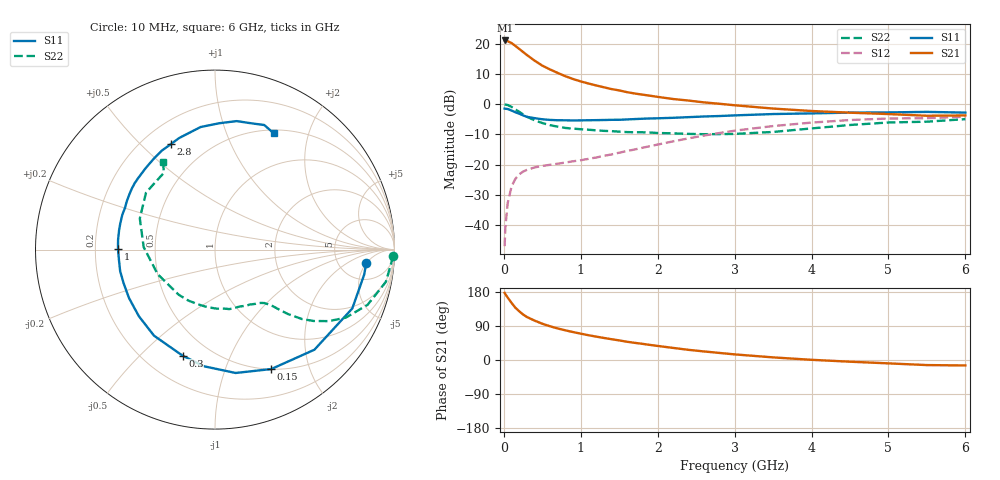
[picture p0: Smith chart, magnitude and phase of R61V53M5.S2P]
! SIEMENS Small Signal Semiconductors
! BFR193
! Si NPN RF Bipolar Junction Transistor in SOT23
! VCE = 1.5 V  IC = 3.5 mA
! Common Emitter S-Parameters:  May  1996
# GHz  S  MA  R  50
!  f  S11  S21  S12  S22
! GHz  MAG  ANG  MAG  ANG  MAG  ANG  MAG  ANG
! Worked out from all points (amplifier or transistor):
!   36 points, 10 MHz to 6 GHz, reference 50 ohm
!   highest |S21| = 21.1 dB at 20 MHz (marker M1)
!   |S21| within 3 dB of that: start of sweep to 209.9 MHz
!   unconditionally stable (mu >= 1): 985.2 MHz to 2.083 GHz
!   at 250 MHz: K = 0.34, MSG = 19.8 dB, |S12| = -22.3 dB
!   at 1.4 GHz: K = 1.09, MAG = 9.0 dB, |S12| = -16.6 dB
!   at 6 GHz: K = 0.99, MSG = 0.2 dB, |S12| = -4.1 dB
!   S11 on the Smith chart (normalised r, x): 10 MHz: 10, -5; 150 MHz: 0.50, -1.46; 300 MHz: 0.35, -0.68; 1 GHz: 0.30, +0.00; 2.8 GHz: 0.31, +0.62; 6 GHz: 0.54, +1.48
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0.01  0.8466 -4.9  11.2 177.2  0.0045 86.1  0.9935 -2.1
0.02  0.8426 -9.6  11.31 173.6  0.0093 83.6  0.985 -4.3
0.05  0.8323 -23.2  10.99 164.7  0.0232 77.4  0.9688 -10.7
0.1  0.7861 -45.2  10.24 150.8  0.0435 67.3  0.904 -19.9
0.15  0.7356 -64.8  9.208 138.0  0.0584 58.4  0.8214 -27.5
0.2  0.697 -80.5  8.195 128.6  0.0693 52.5  0.7479 -32.2
0.25  0.6529 -95.4  7.3 120.1  0.0769 47.9  0.6784 -35.9
0.3  0.6179 -107.0  6.499 113.5  0.0821 44.9  0.6202 -38.6
0.4  0.5878 -125.3  5.244 103.9  0.0902 41.6  0.5409 -41.5
0.5  0.5636 -138.8  4.342 95.7  0.0954 40.2  0.4883 -43.1
0.6  0.55 -150.5  3.756 89.0  0.0996 40.4  0.4501 -44.4
0.7  0.5426 -159.7  3.289 83.2  0.1038 41.5  0.425 -45.8
0.8  0.5419 -167.2  2.901 78.3  0.1085 42.9  0.4052 -47.3
1  0.5405 179.5  2.378 69.5  0.1184 46.2  0.3861 -50.5
1.1  0.5428 174.2  2.198 65.4  0.1249 48.0  0.3781 -53.0
1.6  0.5597 151.6  1.583 48.2  0.1682 55.3  0.346 -66.4
2.2  0.5959 130.5  1.218 31.9  0.2431 56.3  0.3295 -88.2
2.8  0.6372 112.6  1.017 18.7  0.3334 50.7  0.3205 -117.7
3.5  0.6876 96.7  0.847 6.9  0.4351 39.2  0.3477 -156.9
4.5  0.7261 80.4  0.724 -4.5  0.5472 21.2  0.4534 157.5
5.5  0.7464 68.4  0.644 -13.4  0.5873 3.8  0.5138 123.7
6  0.7263 63.3  0.652 -14.4  0.6219 -1.1  0.5667 120.7
